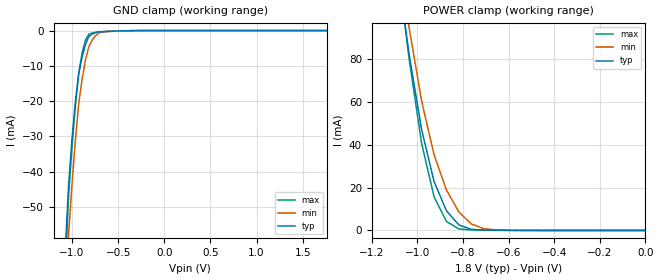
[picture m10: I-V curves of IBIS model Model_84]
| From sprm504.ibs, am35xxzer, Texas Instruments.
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| Model based on original model for IQ1833DVTPBFZP18LL_7LM
|   Sub model PBFZP18LL_7LM_PI_1P8
[model]   Model_84
|[Description]  1.8V-INPUT-PI-X
|[Input Load]   PI
|[Output Drive]
|Voltage   1.8V
|Mode   INPUT
Model_type   Input
Polarity   Non-Inverting
Vinl =  0.63V
Vinh =  1.17V
C_comp   1.254226p   1.200533p   1.264851p
[Model Spec]
Vinl   0.63V   0.567V   0.693V
Vinh   1.17V   1.053V   1.287V
[Temperature Range]   25   125   -40
[Voltage Range]   1.8   1.62   1.98
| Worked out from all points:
|   GND clamp passes 1 mA (typ) near -0.78 V on its own axis
|   POWER clamp passes 1 mA (typ) near -0.78 V on its own axis
[POWER_clamp]
-1.8V     812.4mA    848.7mA    874.6mA
-1.055V   95.91mA    108mA      95.46mA
-1.036V   81.87mA    94.3mA     79.67mA
-1.018V   70.24mA    82.96mA    66.66mA
-981.8mV  46.97mA    60.28mA    40.62mA
-927.3mV  22.83mA    35.31mA    15.72mA
-872.7mV  9.161mA    18.85mA    4.186mA
-818.2mV  2.574mA    8.576mA    711.8uA
-763.6mV  549.3uA    3.016mA    234.2uA
-709.1mV  168.6uA    853.8uA    154.4uA
-654.5mV  89.89uA    236.3uA    110.4uA
0V        17.58nA    52.35nA    29.19nA
[GND_clamp]
-1.8V     -593.4mA   -494.6mA   -853.3mA
-1.073V   -62.13mA   -74.14mA   -68.26mA
-1.036V   -43.76mA   -57.65mA   -46.65mA
-1V       -30.75mA   -43.64mA   -33.1mA
-963.6mV  -20.27mA   -31.35mA   -21.56mA
-927.3mV  -12.32mA   -20.76mA   -12.03mA
-890.9mV  -7.558mA   -13.89mA   -6.391mA
-854.5mV  -4.019mA   -8.509mA   -2.715mA
-818.2mV  -1.706mA   -4.609mA   -1.003mA
-745.5mV  -545.1uA   -1.421mA   -528.1uA
-600mV    -195.8uA   -181.2uA   -256.1uA
1.764V    17.33nA    69.31nA    24.84nA
